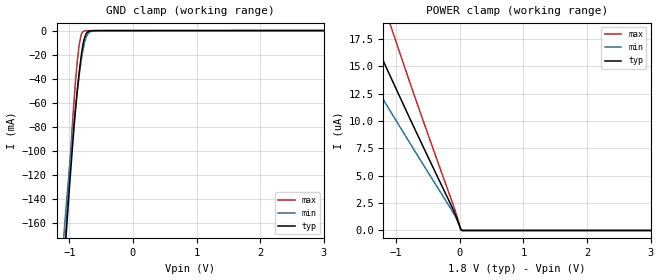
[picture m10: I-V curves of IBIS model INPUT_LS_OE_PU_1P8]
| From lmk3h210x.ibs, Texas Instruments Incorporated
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[Model]   INPUT_LS_OE_PU_1P8
Model_type   Input
Vinl = 0.65
Vinh = 1.15
|   typ   min   max
C_comp   0.7pF   0.5pF   0.9pF
[Voltage Range]   1.8   1.71   1.89
[Temperature Range]   45   125   -40
[Power Clamp Reference]   1.8   1.71   1.89
[GND Clamp Reference]   0   0   0
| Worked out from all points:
|   GND clamp passes 1 mA (typ) near -0.71 V on its own axis
[GND Clamp]
|   Voltage   I(typ)   I(min)   I(max)
-3.3V     -2.163A    -1.946A    -2.393A
-1.142V   -244.3mA   -209.2mA   -247.1mA
-1.073V   -188.3mA   -161.6mA   -183.1mA
-1.043V   -165mA     -142.3mA   -156.4mA
-943.8mV  -92.72mA   -84.36mA   -72.67mA
-874.5mV  -50.36mA   -50.22mA   -25.72mA
-844.8mV  -35.2mA    -37.39mA   -12.04mA
-815.1mV  -22.25mA   -25.97mA   -4.072mA
-765.6mV  -7.258mA   -11.33mA   -432.8uA
-696.3mV  -705.7uA   -2.056mA   -63.37uA
-577.5mV  -41.35uA   -100.4uA   -46.86uA
6.6V      0A         0A         0A
[POWER Clamp]
|   Voltage   I(typ)   I(min)   I(max)
-3.3V     44.5uA     33.74uA    61.67uA
-1.835V   23.76uA    18.2uA     32.15uA
-1.488V   19.2uA     14.77uA    25.82uA
-1.162V   14.99uA    11.59uA    20.02uA
-815.1mV  10.62uA    8.289uA    14.06uA
-498.3mV  6.718uA    5.317uA    8.777uA
-82.5mV   1.636uA    1.4uA      1.994uA
-33mV     920.3nA    816.8nA    1.085uA
16.5mV    95.06nA    157.4nA    27.34nA
26.4mV    47.53nA    30.27nA    13.67nA
46.2mV    0A         0A         0A
6.6V      0A         0A         0A
